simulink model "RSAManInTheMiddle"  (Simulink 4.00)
settings: Solver=ode45  StartTime=0.0  StopTime=10.0  RelTol=1e-3

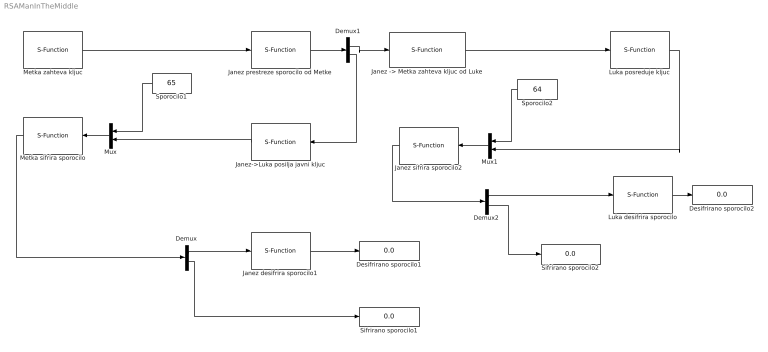
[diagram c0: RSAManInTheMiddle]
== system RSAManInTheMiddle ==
  Demux : Demux  Outputs=2  BusSelectionMode=off
  Demux1 : Demux  Outputs=2  BusSelectionMode=off
  Demux2 : Demux  Outputs=2  BusSelectionMode=off
  Desifrirano sporocilo1 : Display
  Desifrirano sporocilo2 : Display
  "Janez -> Metka zahteva kljuc od Luke" : S-Function  FunctionName=napad_pridobiKljuc  PortCounts=[]  SFunctionModules=''
  Janez desifrira sporocilo1 : S-Function  FunctionName=desifrirajSporocilo  Parameters=37,527  PortCounts=[]  SFunctionModules=''
  Janez prestreze sporocilo od Metke : S-Function  FunctionName=prestreziSporocilo  PortCounts=[]  SFunctionModules=''
  Janez sifrira sporocilo2 : S-Function  Orientation=left  FunctionName=sifrirajSporocilo  PortCounts=[]  SFunctionModules=''
  Janez->Luka posilja javni kljuc : S-Function  Orientation=left  FunctionName=posredujKljuc  Parameters=13,527  PortCounts=[]  SFunctionModules=''
  Luka desifrira sporocilo : S-Function  FunctionName=desifrirajSporocilo  Parameters=37,527  PortCounts=[]  SFunctionModules=''
  Luka posreduje kljuc : S-Function  FunctionName=posredujKljuc  Parameters=13,527  PortCounts=[]  SFunctionModules=''
  Metka sifrira sporocilo : S-Function  Orientation=left  FunctionName=sifrirajSporocilo  PortCounts=[]  SFunctionModules=''
  Metka zahteva kljuc : S-Function  FunctionName=pridobiKljuc  PortCounts=[]  SFunctionModules=''
  Mux : Mux  Orientation=left  Inputs=2
  Mux1 : Mux  Orientation=left  Inputs=2
  Sifrirano sporocilo1 : Display
  Sifrirano sporocilo2 : Display
  Sporocilo1 : Constant  Orientation=left  Value=65
  Sporocilo2 : Constant  Orientation=left  Value=64
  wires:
  Luka desifrira sporocilo/1 -> Desifrirano sporocilo2/1
  Metka sifrira sporocilo/1 -> Demux/1
  Sporocilo1/1 -> Mux/1
  Mux/1 -> Metka sifrira sporocilo/1
  Demux/2 -> Sifrirano sporocilo1/1
  Metka zahteva kljuc/1 -> Janez prestreze sporocilo od Metke/1
  "Janez -> Metka zahteva kljuc od Luke"/1 -> Luka posreduje kljuc/1
  Janez prestreze sporocilo od Metke/1 -> Demux1/1
  Demux1/1 -> "Janez -> Metka zahteva kljuc od Luke"/1
  Demux1/2 -> Janez->Luka posilja javni kljuc/1
  Janez->Luka posilja javni kljuc/1 -> Mux/2
  Demux/1 -> Janez desifrira sporocilo1/1
  Janez desifrira sporocilo1/1 -> Desifrirano sporocilo1/1
  Mux1/1 -> Janez sifrira sporocilo2/1
  Sporocilo2/1 -> Mux1/1
  Luka posreduje kljuc/1 -> Mux1/2
  Janez sifrira sporocilo2/1 -> Demux2/1
  Demux2/1 -> Luka desifrira sporocilo/1
  Demux2/2 -> Sifrirano sporocilo2/1
